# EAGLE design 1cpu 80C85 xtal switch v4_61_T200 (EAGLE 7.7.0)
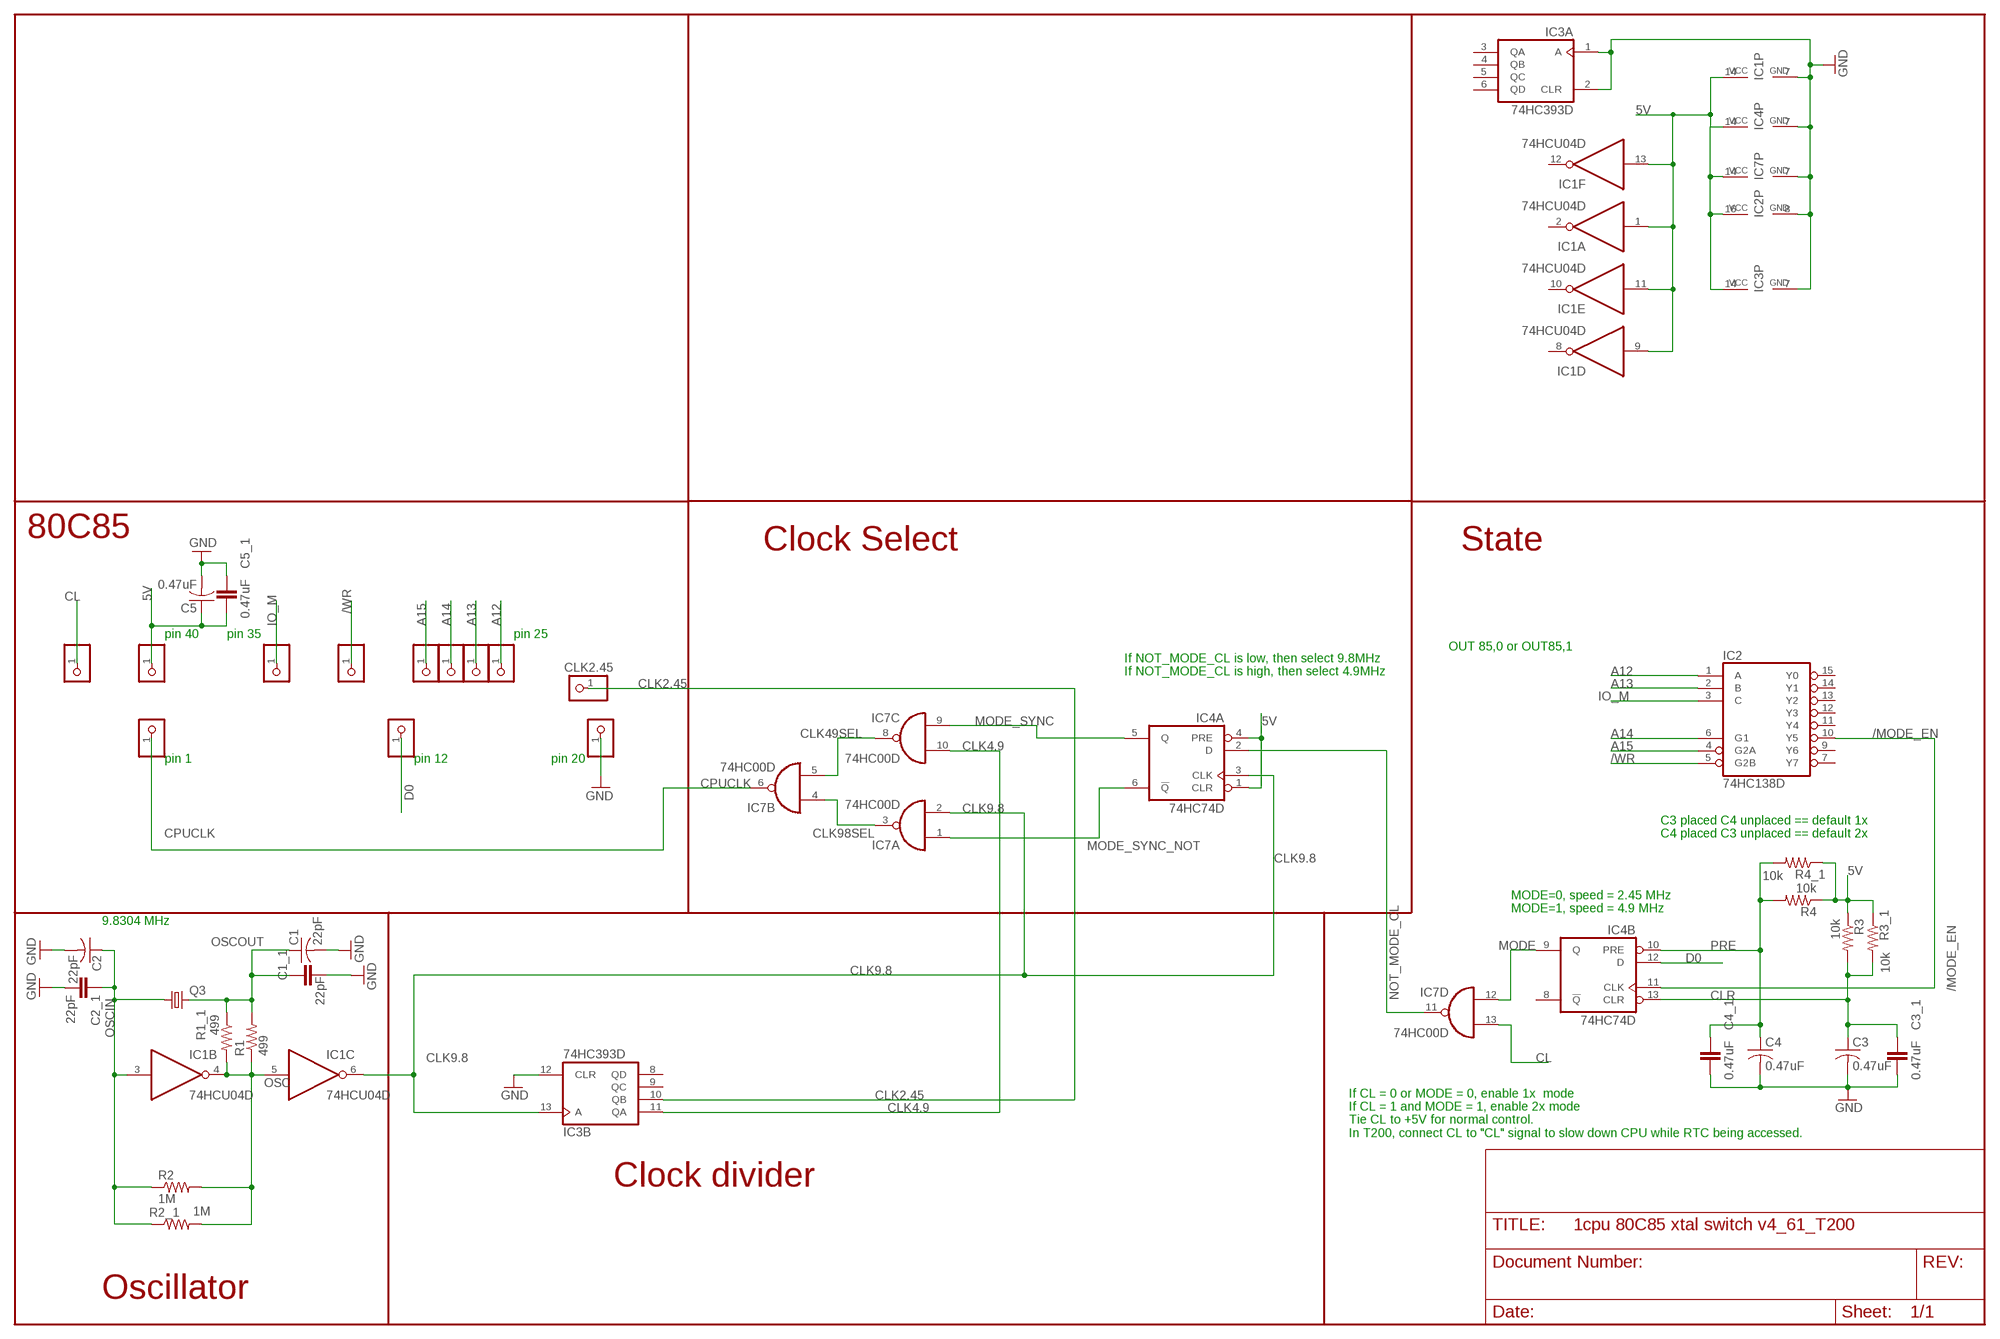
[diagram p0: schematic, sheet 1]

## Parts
5V  PINHD-1X1  [1X01]
5V1  PINHD-1X1  [1X01]
5V2  PINHD-1X1  [1X01]
5V3  PINHD-1X1  [1X01]
5V7  PINHD-1X1  [1X01]
5V8  PINHD-1X1  [1X01]
5V9  PINHD-1X1  [1X01]
5V10  PINHD-1X1  [1X01]
C1  22pF  C-US025-025X050  [C025-025X050]
C1_1  22pF  CAP0805  [0805]
C2  22pF  C-US025-025X050  [C025-025X050]
C2_1  22pF  CAP0805  [0805]
C3  0.47uF  C-US025-025X050  [C025-025X050]
C3_1  0.47uF  CAP0805  [0805]
C4  0.47uF  C-US025-025X050  [C025-025X050]
C4_1  0.47uF  CAP0805  [0805]
C5  0.47uF  C-US025-025X050  [C025-025X050]
C5_1  0.47uF  CAP0805  [0805]
CL  PINHD-1X1  [1X01]
GND5  PINHD-1X1  [1X01]
GND8  PINHD-1X1  [1X01]
IC1  74HCU04D  74HC04D  [SO14]
IC2  74HC138D  [SO16]
IC3  74HC393D  [SO14]
IC4  74HC74D  [SO14]
IC7  74HC00D  [SO14]
Q3  CRYSTALHC49S  [HC49/S]
R1  499  R-US_0204/5  [0204/5]
R1_1  499  RESISTOR0805  [0805]
R2  1M  R-US_0204/5  [0204/5]
R2_1  1M  RESISTOR0805  [0805]
R3  10k  R-US_0204/5  [0204/5]
R3_1  10k  RESISTOR0805  [0805]
R4  10k  R-US_0204/5  [0204/5]
R4_1  10k  RESISTOR0805  [0805]
SEL2  PINHD-1X1  [1X01]

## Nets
5V: 5V.1 C5.1 C5_1.2 IC1.1(A:I) IC1.9(D:I) IC1.11(E:I) IC1.13(F:I) IC1.14(P:VCC) IC2.16(VCC) IC3.14(P:VCC) IC4.1(A:CLR) IC4.4(A:PRE) IC4.14(P:VCC) IC7.14(P:VCC) R3.1 R3_1.1 R4.1 R4_1.1
/MODE_EN: IC2.10(Y5) IC4.11(B:CLK)
/WR: 5V3.1 IC2.5(G2B)
A12: 5V10.1 IC2.1(A)
A13: 5V9.1 IC2.2(B)
A14: 5V8.1 IC2.6(G1)
A15: 5V7.1 IC2.4(G2A)
CL: CL.1 IC7.13(D:I1)
CLK2.45: IC3.10(B:QB) SEL2.1
CLK4.9: IC3.11(B:QA) IC7.10(C:I1)
CLK9.8: IC1.6(C:O) IC3.13(B:A) IC4.3(A:CLK) IC7.2(A:I1)
CLK49SEL: IC7.5(B:I1) IC7.8(C:O)
CLK98SEL: IC7.3(A:O) IC7.4(B:I0)
CLR: C3.1 C3_1.1 IC4.13(B:CLR) R3.2 R3_1.2
CPUCLK: 5V2.1 IC7.6(B:O)
D0: GND8.1 IC4.12(B:D)
GND: C1.2 C1_1.1 C2.2 C2_1.1 C3.2 C3_1.2 C4.2 C4_1.2 C5.2 C5_1.1 GND5.1 IC1.7(P:GND) IC2.8(GND) IC3.1(A:A) IC3.2(A:CLR) IC3.7(P:GND) IC3.12(B:CLR) IC4.7(P:GND) IC7.7(P:GND)
IO_M: 5V1.1 IC2.3(C)
MODE: IC4.9(B:Q) IC7.12(D:I0)
MODE_SYNC: IC4.5(A:Q) IC7.9(C:I0)
MODE_SYNC_NOT: IC4.6(A:!Q) IC7.1(A:I0)
NOT_MODE_CL: IC4.2(A:D) IC7.11(D:O)
OSC: IC1.4(B:O) IC1.5(C:I) R1.1 R1_1.2 R2.2 R2_1.2
OSCIN: C2.1 C2_1.2 IC1.3(B:I) Q3.1 R2.1 R2_1.1
OSCOUT: C1.1 C1_1.2 Q3.2 R1.2 R1_1.1
PRE: C4.1 C4_1.1 IC4.10(B:PRE) R4.2 R4_1.2
Unconnected: IC1.2(A:O) IC1.8(D:O) IC1.10(E:O) IC1.12(F:O) IC2.7(Y7) IC2.9(Y6) IC2.11(Y4) IC2.12(Y3) IC2.13(Y2) IC2.14(Y1) IC2.15(Y0) IC3.3(A:QA) IC3.4(A:QB) IC3.5(A:QC) IC3.6(A:QD) IC3.8(B:QD) IC3.9(B:QC) IC4.8(B:!Q)

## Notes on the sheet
- 80C85
- Clock Select | State
- pin 40 | pin 35 | pin 25
- OUT 85,0 or OUT85,1
- If NOT_MODE_CL is low, then select 9.8MHz
  If NOT_MODE_CL is high, then select 4.9MHz
- pin 1 | pin 12 | pin 20
- C3 placed C4 unplaced == default 1x
  C4 placed C3 unplaced == default 2x
- MODE=0, speed = 2.45 MHz
  MODE=1, speed = 4.9 MHz
- 9.8304 MHz
- If CL = 0 or MODE = 0, enable 1x  mode
  If CL = 1 and MODE = 1, enable 2x mode
  Tie CL to +5V for normal control.
  In T200, connect CL to "CL" signal to slow down CPU while RTC being accessed.
- Clock divider
- Oscillator

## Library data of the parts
5V 5V1-5V3 5V7-5V10 CL GND5 GND8 SEL2 = pinhead:PINHD-1X1: PIN HEADER
C1-C5 = resistor:C-US: CAPACITOR, American symbol
C1_1 C2_1 C3_1 C4_1 C5_1 = SparkFun:CAP: Capacitor
IC1 = 74xx-eu:74*04: Hex INVERTER
IC2 = 74xx-eu:74*138: 3-line to 8-line DECODER/DEMULTIPLEXER
IC3 = 74xx-eu:74*393: Dual 4-bit decade and binary COUNTER
IC4 = 74xx-eu:74*74: Dual D type positive edge triggered FLIP FLOP, preset and clear
IC7 = 74xx-eu:74*00: Quad 2-input NAND gate
Q3 = crystal:CRYSTAL: CRYSTAL; OC_FARNELL: 1667008; OC_NEWARK: unknown
R1-R4 = resistor:R-US_: RESISTOR, American symbol
R1_1 R2_1 R3_1 R4_1 = SparkFun-Resistors:RESISTOR: Generic Resistor Package

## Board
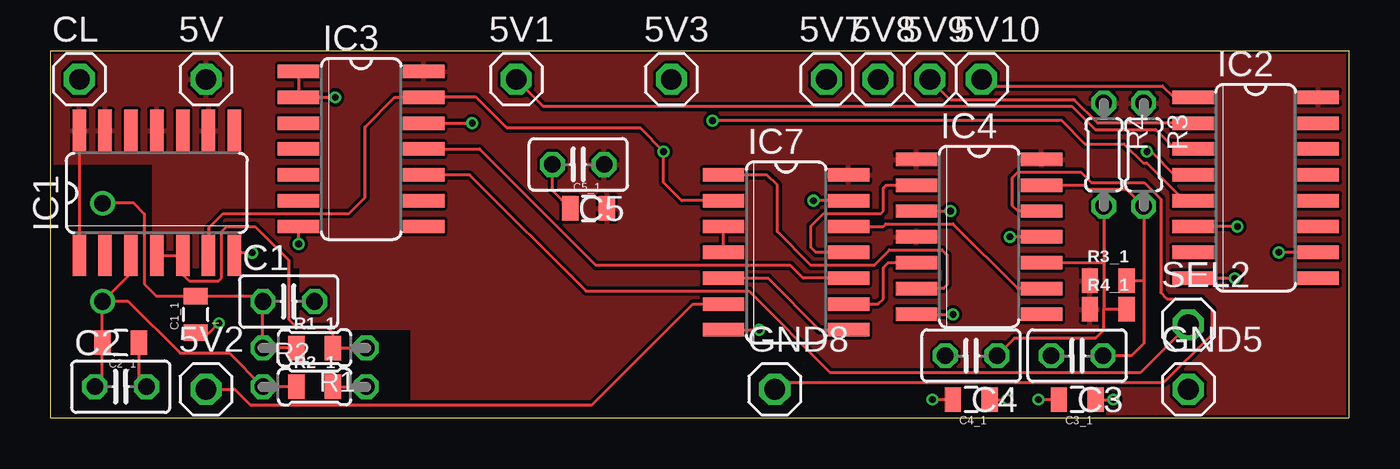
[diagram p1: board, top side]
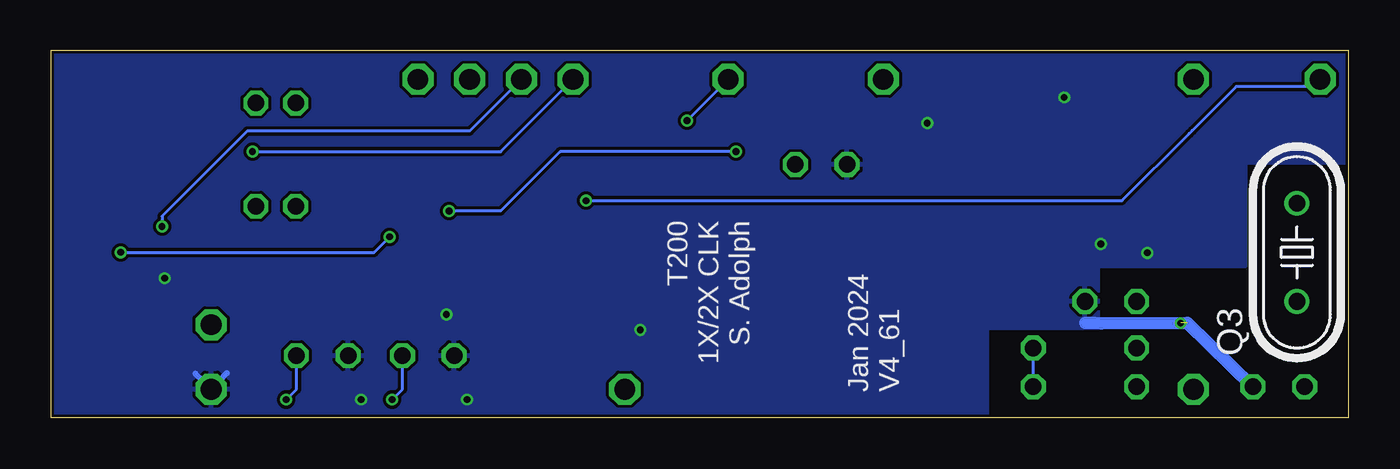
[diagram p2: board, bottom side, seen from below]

Size 63.75 x 18.03 mm. Coordinates in mm from the lower left corner, seen from the top.
Outline: 0,0 63.75,0 63.75,18.03 0,18.03 0,0
Copper layers (1*16): Top 0.035559375mm / dielectric 1.6mm / Bottom 0.035559375mm
Design rules "oshpark-2layer *": minimum track width 6mil, minimum drill 10mil, track to track 6mil, track to pad 6mil, pad to pad 6mil, via to via 6mil, smd to smd 6mil, copper to edge 6mil, drill to drill 6mil, minimum pad ring 5mil, minimum via ring 5mil, stop-mask expansion 2.5mil, vias tented up to drill 0mil, thermal gap 6mil

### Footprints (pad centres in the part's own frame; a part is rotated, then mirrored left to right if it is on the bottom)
1X01 = drill 1.016 octagon: 1 0,0
C025-025X050 = drill 0.813 octagon: 1 -1.27,0; 2 1.27,0
0805 = smd 0.8 x 1.2: 1 -0.9,0; 2 0.9,0
SO14 = smd 0.66 x 2.032: 1 -3.81,-3.073; 2 -2.54,-3.073; 3 -1.27,-3.073; 4 0,-3.073; 5 1.27,-3.073; 6 2.54,-3.073; 7 3.81,-3.073; 8 3.81,3.073; 9 2.54,3.073; 10 1.27,3.073; 11 0,3.073; 12 -1.27,3.073; 13 -2.54,3.073; 14 -3.81,3.073
SO16 = smd 0.66 x 2.032: 1 -4.445,-3.073; 2 -3.175,-3.073; 3 -1.905,-3.073; 4 -0.635,-3.073; 5 0.635,-3.073; 6 1.905,-3.073; 7 3.175,-3.073; 8 4.445,-3.073; 9 4.445,3.073; 10 3.175,3.073; 11 1.905,3.073; 12 0.635,3.073; 13 -0.635,3.073; 14 -1.905,3.073; 15 -3.175,3.073; 16 -4.445,3.073
HC49/S = drill 0.813: 1 -2.413,0; 2 2.413,0
0204/5 = drill 0.813 octagon: 1 -2.54,0; 2 2.54,0

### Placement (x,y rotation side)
5V  7.62,16.64 0 top
5V1  22.86,16.64 0 top
5V2  7.62,1.4 0 top
5V3  30.48,16.64 0 top
5V7  38.1,16.64 0 top
5V8  40.64,16.64 0 top
5V9  43.18,16.64 0 top
5V10  45.72,16.64 0 top
C1  11.68,5.71 0 top
C1_1  7.11,5.08 90 top
C2  3.43,1.52 0 top
C2_1  3.43,3.68 180 top
C3  50.42,3.05 180 top
C3_1  50.42,0.89 180 top
C4  45.21,3.05 180 top
C4_1  45.21,0.89 180 top
C5  25.91,12.45 180 top
C5_1  26.42,10.29 0 top
CL  1.4,16.64 0 top
GND5  55.88,1.4 0 top
GND8  35.56,1.4 0 top
IC1  5.21,11.05 0 top
IC2  59.18,11.3 270 top
IC3  15.24,13.21 270 top
IC4  45.59,8.89 270 top
IC7  36.12,8.13 270 top
Q3  2.54,8.13 90 bottom
R1  12.95,3.43 180 top
R1_1  12.95,3.43 0 top
R2  12.95,1.52 0 top
R2_1  12.95,1.52 0 top
R3  53.68,12.93 270 top
R3_1  51.94,6.73 0 top
R4  51.73,12.93 270 top
R4_1  51.94,5.33 0 top
SEL2  55.88,4.57 0 top

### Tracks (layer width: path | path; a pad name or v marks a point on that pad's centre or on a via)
5V
  Top 0.152: IC1.14 IC1.1
  pour Top: 0.08,17.96 0.08,12.52 5.03,12.52 5.03,7.44 12.27,7.44 12.27,4.39 17.73,4.39 17.73,0.08 63.68,0.08 63.68,17.96
/MODE_EN  (via drill 0.33)
  Top 0.152: IC4.11 v47.12,8.89 | IC2.10 v60.33,8.13
  Bottom 0.152: v47.12,8.89 47.88,8.13 v60.33,8.13
/WR  (via drill 0.33)
  Top 0.152: v32.5,14.61 49.66,14.61 50.8,13.46 52.72,13.46 53.66,12.52 53.84,12.52 55.69,10.67 IC2.5
  Bottom 0.152: 5V3.1 30.48,16.62 v32.5,14.61
A12
  Top 0.152: 5V10.1 46.05,16.31 54.61,16.31 55.17,15.75 IC2.1
A13
  Top 0.152: IC2.2 51.44,14.48 50.29,15.62 44.2,15.62 5V9.1
A14  (via drill 0.33)
  Top 0.152: v58.29,9.4 IC2.6
  Bottom 0.152: 5V8.1 43.18,14.1 54.1,14.1 58.29,9.91 v58.29,9.4
A15  (via drill 0.33)
  Top 0.152: IC2.4 55.19,11.94 54.05,13.08 v53.85,13.08
  Bottom 0.152: 5V7.1 41.66,13.08 v53.85,13.08
CL  (via drill 0.33)
  Top 0.152: IC7.13 v37.47,10.67
  Bottom 0.152: CL.1 1.75,16.28 5.52,16.28 7.69,14.12 7.84,13.97 11.14,10.67 v37.47,10.67
CLK2.45
  Top 0.152: SEL2.1 53.52,2.21 38.3,2.21 34.29,6.22 26.29,6.22 20.57,11.94 IC3.10
CLK4.9
  Top 0.152: IC7.10 36.96,6.86 36.32,7.49 26.78,7.49 21.07,13.21 IC3.11
CLK9.8  (via drill 0.33)
  Top 0.152: IC1.6 7.77,8.13 7.77,8.62 7.75,8.65 7.75,9.32 8.46,10.03 14.64,10.03 15.43,10.82 15.43,14.29 16.89,15.75 IC3.13 18.33,15.76 20.88,15.76 22.42,14.22 28.96,14.22 v30.1,13.08 30.1,11.56 30.99,10.67 IC7.2 | IC4.3 v44.2,10.16
  Bottom 0.152: v30.1,13.08 38.73,13.08 41.66,10.16 v44.2,10.16
CLK49SEL
  Top 0.152: IC7.5 35.23,6.86 37.77,4.32 IC7.8
CLK98SEL
  Top 0.152: IC7.4 IC7.3
CLR  (via drill 0.33)
  Top 0.152: IC4.13 50.79,11.43 50.98,11.24 52.83,11.24 R3.2 53.68,6.74 | 53.68,6.74 53.68,3.65 53.09,3.05 C3.1 | R3_1.2 52.86,6.74 53.68,6.74 | C3_1.1 v52.2,0.89
  Bottom 0.152: v52.2,0.89 51.69,1.4 C3.1
CPUCLK
  Top 0.152: 5V2.1 9.02,1.4 9.78,0.64 26.59,0.64 31.55,5.59 IC7.6
D0
  Top 0.152: GND8.1 35.89,1.73 54.67,1.73 57.02,4.08 57.02,5.33 56.52,5.84 54.83,5.84 54.52,6.15 54.52,10.74 53.71,11.56 51.12,11.56 50.61,12.06 47.5,12.06 47.24,11.81 47.24,10.41 47.5,10.16 IC4.12
GND  (via drill 0.33)  (1 unrouted)
  Top 0.152: IC4.7 v44.32,5.08 | IC7.7 v34.8,4.32 | IC2.8 v58.17,6.86 | IC3.1 IC3.2 v13.97,15.75 | v12.17,8.53 IC3.7 | IC3.12 v20.7,14.48 | v9.89,8.1 9.14,8.1 IC1.7 | C2.2 4.33,1.89 C2_1.1 | C1_1.1 7.79,4.18 v8.25,4.65 | C5_1.1 24.64,11.16 C5.2 | C3_1.2 v48.51,0.89 | C4_1.2 v43.31,0.89
  Bottom 0.152: v34.8,4.32 34.96,4.32 34.96,4.33 | v58.17,6.86 58.03,6.86
  Bottom 0.305: 55.88,1.44 56.64,2.16 | 55.84,1.44 55.12,2.2
  Bottom 0.61: 12.14,4.64 12.94,4.65 12.46,4.65 12.14,4.64 | C2.2 7.92,4.65 12.14,4.64
  pour Bottom: 0.08,17.96 63.68,17.96 63.68,0.08 17.73,0.08 17.73,4.39 12.27,4.39 12.27,7.44 5.03,7.44 5.03,12.52 0.08,12.52
IO_M
  Top 0.152: IC2.3 55.24,13.21 54.28,14.17 51.31,14.17 50.18,15.3 24.19,15.3 5V1.1
MODE
  Top 0.152: IC4.9 47.5,6.35 44.32,9.53 41.02,9.53 40.89,9.4 IC7.12 39.22,9.42
MODE_SYNC
  Top 0.152: IC7.9 40.64,5.59 40.89,5.84 40.89,7.38 41.13,7.62 IC4.5
MODE_SYNC_NOT
  Top 0.152: IC7.1 35.18,11.94 35.69,11.43 35.69,9.14 37.34,7.49 40.42,7.49 41.19,8.26 43.78,8.26 44.03,8 44.03,6.53 43.85,6.35 IC4.6
NOT_MODE_CL
  Top 0.152: IC7.11 37.58,8.13 37.34,8.37 37.34,9.41 37.96,10.03 40.77,10.03 40.89,10.16 40.89,11.29 41.03,11.43 IC4.2
OSC
  Top 0.152: IC1.4 IC1.5 6.48,7.04 6.8,6.72 8.24,6.72 8.38,6.86 8.38,9.14 8.64,9.4 10.03,9.4 11.68,7.75 11.68,4.83 12.07,4.45 13.59,4.45 13.84,4.19 R1_1.2 R1.1 | R2_1.2 R2.2
  Bottom 0.152: R2.2 R1.1
OSCIN
  Top 0.152: IC1.3 3.94,7.11 Q3.1 | C2.1 2.53,1.89 C2_1.2 Q3.1 | R2_1.1 R2.1 8.76,3.17 6.35,3.17 3.81,5.71 Q3.1
OSCOUT
  Top 0.152: Q3.2 4.06,10.54 4.58,10.02 4.58,6.58 5.18,5.98 C1_1.2 10.15,5.98 C1.1 R1.2 R1_1.1
PRE  (via drill 0.33)
  Top 0.152: C4.1 47.33,3.9 51.31,3.9 51.73,4.32 51.73,5.33 | R4.2 51.73,7.59 | 51.73,7.59 51.73,5.33 | IC4.10 51.7,7.62 51.73,7.59 | R4_1.2 51.73,5.33 | C4_1.1 v46.99,0.89
  Bottom 0.152: v46.99,0.89 46.48,1.4 C4.1

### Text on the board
_tsilk: +5 | CL | IO/M | /WR | A15 | A14 | A13 | A12 | 74HCU04 | 74HC393 | C5 | R4 | R3 | 74HC138 | 74HC74 | 74HC00 | R3 | C1 | R4 | 2.45M | C2 | R1 | D0 | 1 | C4 | C3 | GND | R2 | 2X | 1X
_bsilk: T200 / 1X/2X CLK / S. Adolph | Jan 2024 / V4_61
